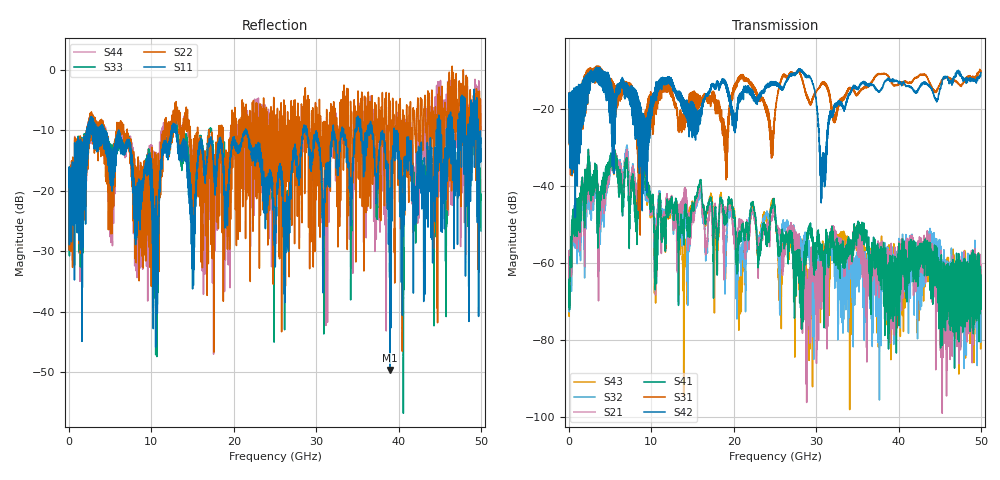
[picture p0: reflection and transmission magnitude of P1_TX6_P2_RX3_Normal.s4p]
!Keysight Technologies,N5225B,MY57041031,A.13.20.10
!Date: Friday, May 31, 2019 11:32:02
!Correction: S11(Full 4 Port(1,2,3,4))
!S12(Full 4 Port(1,2,3,4))
!S13(Full 4 Port(1,2,3,4))
!S14(Full 4 Port(1,2,3,4))
!S21(Full 4 Port(1,2,3,4))
!S22(Full 4 Port(1,2,3,4))
!S23(Full 4 Port(1,2,3,4))
!S24(Full 4 Port(1,2,3,4))
!S31(Full 4 Port(1,2,3,4))
!S32(Full 4 Port(1,2,3,4))
!S33(Full 4 Port(1,2,3,4))
!S34(Full 4 Port(1,2,3,4))
!S41(Full 4 Port(1,2,3,4))
!S42(Full 4 Port(1,2,3,4))
!S43(Full 4 Port(1,2,3,4))
!S44(Full 4 Port(1,2,3,4))
!S4P File: Measurements: <S11,S12,S13,S14>,
!<S21,S22,S23,S24>,
!<S31,S32,S33,S34>,
!<S41,S42,S43,S44>:
# Hz S  dB  R 50.0
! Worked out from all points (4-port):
!   5000 points, 10 MHz to 50 GHz, reference 50 ohm
!   strongest paths, dB at 10 MHz, 12.51 GHz, 25.01 GHz, 37.51 GHz, 50 GHz:
!     S42: -19.3, -14.2, -13.2, -15.1, -10.4
!     S31: -19.2, -15.5, -21.6, -10.8, -9.9
!     S41: -67.1, -43.4, -46.1, -58.8, -63.2
!     S21: -67.0, -44.4, -47.2, -60.5, -66.6
!     S32: -63.0, -44.4, -46.0, -64.5, -67.0
!     S43: -68.3, -44.6, -46.0, -66.4, -65.5
!   lowest |S11| = -49.6 dB at 38.96 GHz (marker M1), VSWR 1.01, Z = 50.3 + j0.199 ohm
!   |S11| at or under -10 dB: 4.286 GHz to 12.47 GHz (8.179 GHz wide, 97.6 % of centre); 13.02 GHz to 21.43 GHz (8.403 GHz wide, 48.8 % of centre); 21.46 GHz to 28.42 GHz (6.96 GHz wide, 27.9 % of centre)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
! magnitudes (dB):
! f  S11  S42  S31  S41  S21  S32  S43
! 10 MHz  -19.4  -19.3  -19.2  -67.1  -67.0  -63.0  -68.3
! 6.98 GHz  -12.5  -16.0  -14.8  -32.5  -30.5  -29.6  -30.8
! 14.12 GHz  -14.6  -18.4  -19.4  -44.7  -40.5  -42.4  -53.8
! 28.09 GHz  -13.9  -9.6  -11.0  -59.7  -62.2  -58.3  -54.5
! 30.78 GHz  -22.6  -33.3  -13.3  -57.0  -65.8  -61.9  -57.4
! 38.96 GHz  -49.6  -12.8  -12.3  -67.5  -58.6  -58.3  -60.9
! 50 GHz  -11.3  -10.4  -9.9  -63.2  -66.6  -67.0  -65.5
